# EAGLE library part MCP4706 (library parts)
MCP4706 I2C DAC
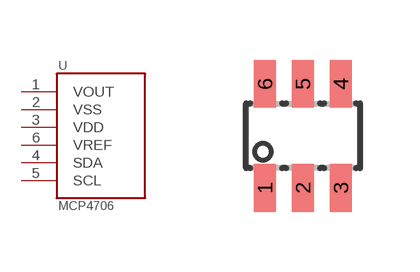
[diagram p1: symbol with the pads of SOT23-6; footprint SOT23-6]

Designator prefix -

## MCP4706  [SOT23-6]
1  VOUT
2  VSS
3  VDD
4  SDA
5  SCL
6  VREF

## Footprint SOT23-6 (pad centres in mm)
smd 0.55 x 1.2: 1 -0.95,-1.3; 2 0,-1.3; 3 0.95,-1.3; 4 0.95,1.3; 5 0,1.3; 6 -0.95,1.3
